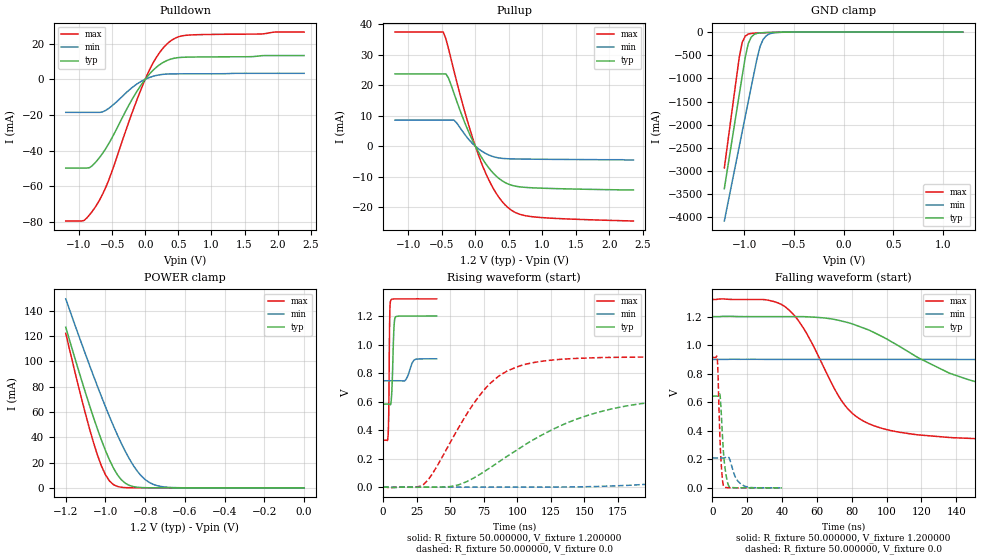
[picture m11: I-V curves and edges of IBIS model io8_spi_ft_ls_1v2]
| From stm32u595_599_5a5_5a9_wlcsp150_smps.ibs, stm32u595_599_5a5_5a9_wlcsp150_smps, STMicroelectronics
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|   Model io8_spi_ft_ls_1v2
[Model]  io8_spi_ft_ls_1v2
Model_type I/O
Polarity   Non-Inverting
Enable   Active-Low
Vinl =   0.360000V
Vinh =   0.840000V
Vmeas =  0.600000V
Cref =   50.000000pF
Rref =   100.000000M
Vref =   0.0V
C_comp   3.132800pF   3.069700pF   3.178000pF
[Temperature Range]   25.000000   0.140000k   -40.000000
[Pullup Reference]   1.200000V   0.900000V   1.320000V
[Pulldown Reference]   0.0V   0.0V   0.0V
[POWER Clamp Reference]   1.200000V   0.900000V   1.320000V
[GND Clamp Reference]   0.0V   0.0V   0.0V
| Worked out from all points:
|   slope of the pulldown table from 0 to 0.18 V, typ, clamps not added: 25.4 ohm
|   slope of the pullup table from 0 to 0.18 V, typ, clamps not added: 27.8 ohm
|   GND clamp passes 1 mA (typ) near -0.51 V on its own axis
|   POWER clamp passes 1 mA (typ) near -0.86 V on its own axis
|   rising waveform, R_fixture 50.000000, V_fixture 1.200000: 20-80 % time 1.25ns typ, 3.35ns min, 598ps max; typ from 0.582 V to 1.2 V
|   rising waveform, R_fixture 50.000000, V_fixture 0.0: 20-80 % time 77.8ns typ, 193ns min, 37.8ns max; typ from 0 V to 0.643 V
|   falling waveform, R_fixture 50.000000, V_fixture 1.200000: 20-80 % time 69.8ns typ, 186ns min, 27.7ns max; typ from 1.2 V to 0.582 V
|   falling waveform, R_fixture 50.000000, V_fixture 0.0: 20-80 % time 2.25ns typ, 4.29ns min, 1.61ns max; typ from 0.643 V to 0 V
[Pulldown]
|Voltage   I(typ)   I(min)   I(max)
-1.2V     -49.85mA   -18.57mA   -79.56mA
-920mV    -49.85mA   -18.57mA   -79.19mA
-840mV    -49.59mA   -18.57mA   -76.08mA
-720mV    -45.32mA   -18.57mA   -69.74mA
-560mV    -36.71mA   -16.58mA   -57.44mA
-200mV    -11.43mA   -4.739mA   -19.03mA
0V        0A         -600fA     0A
160mV     6.476mA    2.074mA    11.78mA
360mV     10.99mA    2.988mA    20.81mA
480mV     12.07mA    3.052mA    23.52mA
640mV     12.43mA    3.073mA    24.76mA
2.4V      13.31mA    3.339mA    26.51mA
[Pullup]
|Voltage   I(typ)   I(min)   I(max)
-1.2V     23.7mA     8.568mA    37.41mA
-480mV    23.7mA     8.568mA    37.41mA
-440mV    23.7mA     8.568mA    35.14mA
-400mV    22.24mA    8.568mA    31.81mA
-320mV    17.36mA    8.568mA    24.69mA
-120mV    5.681mA    2.787mA    8.394mA
80mV      -3.179mA   -1.366mA   -4.88mA
280mV     -9.096mA   -3.48mA    -14.29mA
520mV     -12.61mA   -4.111mA   -20.65mA
680mV     -13.33mA   -4.182mA   -22.38mA
920mV     -13.66mA   -4.239mA   -23.22mA
2.36V     -14.3mA    -4.5mA     -24.47mA
[GND_clamp]
|Voltage   I(typ)   I(min)   I(max)
-1.2V     -3.379A    -4.076A    -2.932A
-1.05V    -1.35A     -2.47A     -550.7mA
-1.02V    -947.8mA   -2.149A    -221.5mA
-990mV    -552.4mA   -1.829A    -88.44mA
-960mV    -255.3mA   -1.51A     -44.87mA
-930mV    -111.8mA   -1.191A    -30.68mA
-870mV    -28.35mA   -564.6mA   -21.34mA
-840mV    -18.65mA   -309.5mA   -18.49mA
-810mV    -14.07mA   -161.6mA   -15.92mA
-780mV    -11.37mA   -83.33mA   -13.53mA
-600mV    -3.009mA   -4.321mA   -3.091mA
1.2V      0A         13.65nA    0A
[POWER_clamp]
|Voltage   I(typ)   I(min)   I(max)
-1.2V     127mA      149.4mA    122.2mA
-1.12V    84.97mA    114mA      70.27mA
-1.06V    55.51mA    88.42mA    35.67mA
-1.02V    37.63mA    72.04mA    17.17mA
-1V       29.51mA    64.13mA    10.3mA
-960mV    15.69mA    48.99mA    2.571mA
-900mV    3.624mA    28.77mA    182.8uA
-840mV    490.7uA    13.24mA    11.35uA
-800mV    116.8uA    6.532mA    1.77uA
-740mV    13.2uA     1.724mA    109.1nA
-620mV    167.4nA    79.36uA    0A
0V        0A         17.87nA    0A
[Ramp]
| variable   typ   min   max
dV/dt_r  0.38562/77.74948n   0.12537/0.19253u   0.54824/37.76723n
dV/dt_f  0.37078/69.71080n   92.19000m/0.18574u  0.59435/27.66254n
R_load = 50.000000
[Rising Waveform]
R_fixture= 50.000000
V_fixture= 1.200000
V_fixture_min= 0.900000
V_fixture_max= 1.320000
|time   V(typ)   V(min)   V(max)
0s        582mV      746mV      329.4mV
3.764ns   582.1mV    746mV      371.6mV
4.244ns   582mV      746mV      556.6mV
4.885ns   579.9mV    746mV      1.177V
5.606ns   579.2mV    746mV      1.307V
6.647ns   707.1mV    746mV      1.318V
8.088ns   1.119V     746mV      1.319V
8.969ns   1.19V      746mV      1.32V
23.06ns   1.2V       891.1mV    1.32V
39.88ns   1.2V       900mV      1.32V
[Rising Waveform]
R_fixture= 50.000000
V_fixture= 0.0
V_fixture_min= 0.0
V_fixture_max= 0.0
|time   V(typ)   V(min)   V(max)
0s        1.999nV    239.3nV    1.184nV
30.03ns   -131.8uV   -196.9uV   17.81mV
56.06ns   15.69mV    -31.47uV   414.2mV
80.08ns   138.1mV    9.383uV    730.3mV
102.1ns   274.9mV    180uV      850.9mV
126.1ns   403.7mV    572.9uV    891.2mV
182.2ns   570.6mV    12.34mV    910.8mV
264.3ns   632.1mV    72.17mV    913.7mV
520.5ns   642.6mV    193.2mV    913.7mV
997ns     642.7mV    209.3mV    913.8mV
[Falling Waveform]
R_fixture= 50.000000
V_fixture= 1.200000
V_fixture_min= 0.900000
V_fixture_max= 1.320000
|time   V(typ)   V(min)   V(max)
0s        1.2V       900mV      1.32V
40.04ns   1.2V       900.1mV    1.282V
52.05ns   1.2V       900mV      1.124V
72.07ns   1.175V     900mV      650.9mV
82.08ns   1.141V     900mV      504.7mV
136.1ns   803.3mV    899.7mV    352.8mV
190.2ns   657.7mV    895.9mV    333.9mV
288.3ns   594.8mV    849.9mV    329.7mV
478.5ns   582.4mV    768.6mV    329.4mV
997ns     582mV      746mV      329.4mV
[Falling Waveform]
R_fixture= 50.000000
V_fixture= 0.0
V_fixture_min= 0.0
V_fixture_max= 0.0
|time   V(typ)   V(min)   V(max)
0s        642.7mV    209.3mV    913.8mV
2.803ns   642.5mV    209.3mV    905.2mV
4.645ns   612.5mV    209.3mV    258.1mV
5.606ns   403.8mV    209mV      79mV
6.486ns   226.3mV    209.2mV    9.465mV
8.168ns   67.02mV    216.1mV    1.806mV
10.01ns   4.382mV    196.1mV    476.6uV
13.53ns   669uV      66.43mV    5.133uV
18.26ns   67.16uV    12.9mV     -57.41uV
39.88ns   1.999nV    239.3nV    1.184nV
